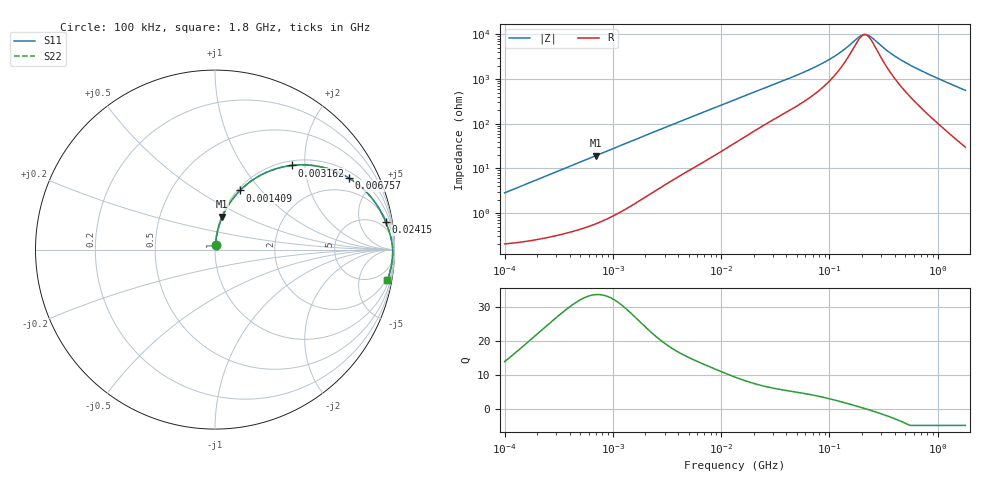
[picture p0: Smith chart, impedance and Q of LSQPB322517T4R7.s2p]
! LSQPB322517T4R7  S-PARAMETER MODEL  ( General Type )
! Model Generated by TAIYO YUDEN Corporation (http://www.ty-top.com)
! Version 2.0
! TAIYO YUDEN Control No. 100810NC14SB-FKC
! Copyright(c) 2008 TAIYO YUDEN CO.,LTD. All Rights Reserved.
! Product Description (link to TY-COMPAS)
! https://ds.yuden.co.jp/TYCOMPAS/or/detail?pn=LSQPB322517T4R7M&u=M
! Products Name : Inductors
! Characteristics :
!  Inductance : 4.7 uH , SRF(min) : 120 MHz , DC Resistance(max) : 0.216 Ohm
!  Rated Current : Saturation :1300 mA , Temp Rise : 1000 mA (40 degC)
!  Case Size : 3.2 x 2.5 / 0.126 x 0.098 [mm/inch] , Thickness : 1.7 / 0.068 [mm/inch]
!  (Conditions: Temperature = 25 degC , DC Bias Current/Voltage = 0A / 0V)
! External Node Assignments :
!  1  o---GGG---o  2
! GND o---------o GND
! Frequency Range : 0.1MHz  -  1800MHz  [ 402 STEP ]
# MHz S RI R 50
! Freq[MHz].  S11 Real  S11 Imag  S21 Real  S21 Imag  S12 Real  S12 Imag  S22 Real  S22 Imag
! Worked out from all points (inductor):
!   401 points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, 100 kHz to 1.8 GHz, reference 50 ohm
!   read as one part in series: L = 4.48 uH near 105 kHz
!   highest Q = 33.6 at 692.5 kHz (marker M1), where L = 4.42 uH
!   self-resonance near 208.5 MHz
!   S11 on the Smith chart (normalised r, x): 100 kHz: 1.00, +0.06; 1.409 MHz: 1.03, +0.78; 3.162 MHz: 1.09, +1.72; 6.757 MHz: 1.27, +3.57; 24.15 MHz: 3, +12; 1.8 GHz: 2, -11
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0.1  0.00282 0.0281  0.9972 -0.0281  0.9972 -0.0281  0.00282 0.0281
0.247521  0.00756 0.0686  0.9924 -0.0686  0.9924 -0.0686  0.00756 0.0686
0.516129  0.0244 0.1394  0.9756 -0.1394  0.9756 -0.1394  0.0244 0.1394
0.692494  0.0407 0.1833  0.9593 -0.1833  0.9593 -0.1833  0.0407 0.1833
1.409041  0.1398 0.3298  0.8602 -0.3298  0.8602 -0.3298  0.1398 0.3298
2.66389  0.3526 0.454  0.6474 -0.454  0.6474 -0.454  0.3526 0.454
3.162158  0.4285 0.4689  0.5715 -0.4689  0.5715 -0.4689  0.4285 0.4689
4.455722  0.5841 0.4624  0.4159 -0.4624  0.4159 -0.4624  0.5841 0.4624
6.757206  0.7466 0.3987  0.2534 -0.3987  0.2534 -0.3987  0.7466 0.3987
9.291023  0.8351 0.3295  0.1649 -0.3295  0.1649 -0.3295  0.8351 0.3295
13.41641  0.9004 0.2504  0.0996 -0.2504  0.0996 -0.2504  0.9004 0.2504
24.15197  0.952 0.1518  0.048 -0.1518  0.048 -0.1518  0.952 0.1518
69.24595  0.9832 0.0542  0.0168 -0.0542  0.0168 -0.0542  0.9832 0.0542
113.0207  0.988 0.0273  0.012 -0.0273  0.012 -0.0273  0.988 0.0273
140.897  0.9891 0.0172  0.0109 -0.0172  0.0109 -0.0172  0.9891 0.0172
184.4683  0.9898 0.00568  0.0102 -0.00568  0.0102 -0.00568  0.9898 0.00568
208.5031  0.99 0.000592  0.00996 -0.000592  0.00996 -0.000592  0.99 0.000592
241.5136  0.9902 -0.00553  0.00983 0.00553  0.00983 0.00553  0.9902 -0.00553
357.3983  0.9899 -0.0229  0.0101 0.0229  0.0101 0.0229  0.9899 -0.0229
467.921  0.9892 -0.0366  0.0108 0.0366  0.0108 0.0366  0.9892 -0.0366
659.3364  0.9872 -0.0581  0.0128 0.0581  0.0128 0.0581  0.9872 -0.0581
1800  0.9606 -0.1698  0.0394 0.1698  0.0394 0.1698  0.9606 -0.1698
